// ------------------------------------------------------------------
// File           : C:\Programmi\Siemens\NCVar Selector\OP40md.awl
//
// Source File    : C:\Programmi\Siemens\NCVar Selector\OP40md.var
// Generation Date: 18/02/2015  Time: 9.30.56
// ------------------------------------------------------------------

DATA_BLOCK DB  121
VERSION : 0.0


STRUCT

 A2_M_POS_LIMIT_PLUS_z:
   STRUCT
   SYNTAX_ID : BYTE  := B#16#82;
   bereich_u_einheit : BYTE := B#16#62;
   spalte : WORD := W#16#8D0E;
   zeile : WORD := W#16#1;
   bausteintyp : BYTE := B#16#1A;
   ZEILENANZAHL : BYTE := B#16#1;
   typ : BYTE := B#16#F;
   laenge : BYTE := B#16#8;
   END_STRUCT ;

 A5_M_POS_LIMIT_MINUS_z2:
   STRUCT
   SYNTAX_ID : BYTE  := B#16#82;
   bereich_u_einheit : BYTE := B#16#65;
   spalte : WORD := W#16#8D04;
   zeile : WORD := W#16#1;
   bausteintyp : BYTE := B#16#1A;
   ZEILENANZAHL : BYTE := B#16#1;
   typ : BYTE := B#16#F;
   laenge : BYTE := B#16#8;
   END_STRUCT ;

 END_STRUCT ;

BEGIN
END_DATA_BLOCK
